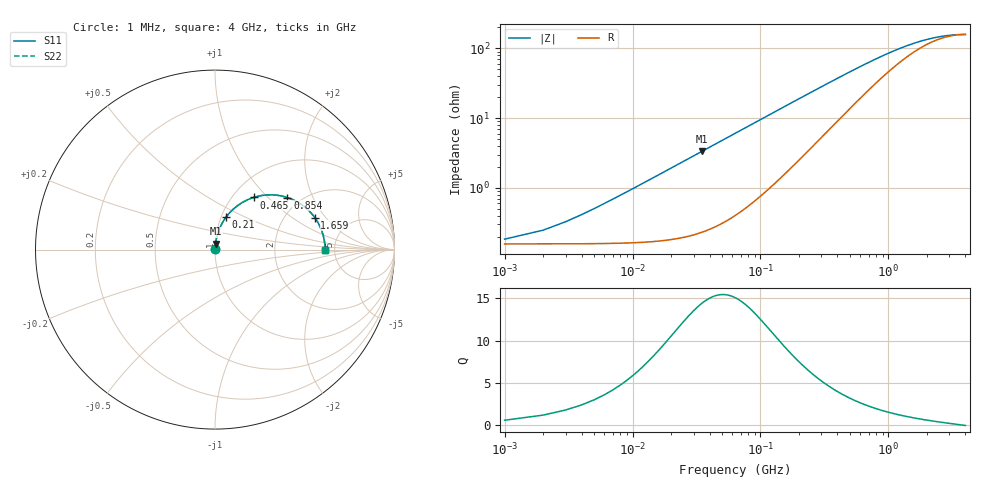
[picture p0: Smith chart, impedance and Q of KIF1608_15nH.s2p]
# MHz S RI R 50
!Freq ReS11 ImS11 ReS21 ImS21 ReS12 ImS12 ReS22 ImS22
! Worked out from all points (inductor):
!   4000 points, 1 MHz to 4 GHz, reference 50 ohm
!   read as one part in series: L = 15.2 nH near 21 MHz
!   highest Q = 14.4 at 35 MHz (marker M1), where L = 15.2 nH
!   self-resonance near 3.966 GHz
!   S11 on the Smith chart (normalised r, x): 1 MHz: 1.00, +0.00; 210 MHz: 1.05, +0.39; 465 MHz: 1.24, +0.83; 854 MHz: 1.71, +1.32; 1.659 GHz: 2.88, +1.56; 4 GHz: 4.17, -0.02
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1  0.00157 0.000954  0.9984 -0.000954  0.9984 -0.000954  0.00157 0.000954
11  0.00175 0.0105  0.9982 -0.0105  0.9982 -0.0105  0.00175 0.0105
24  0.00244 0.0229  0.9976 -0.0229  0.9976 -0.0229  0.00244 0.0229
29  0.00284 0.0276  0.9972 -0.0276  0.9972 -0.0276  0.00284 0.0276
35  0.00342 0.0333  0.9966 -0.0333  0.9966 -0.0333  0.00342 0.0333
46  0.00476 0.0436  0.9952 -0.0436  0.9952 -0.0436  0.00476 0.0436
60  0.00698 0.0567  0.993 -0.0567  0.993 -0.0567  0.00698 0.0567
77  0.0104 0.0723  0.9896 -0.0723  0.9896 -0.0723  0.0104 0.0723
96  0.0152 0.0894  0.9848 -0.0894  0.9848 -0.0894  0.0152 0.0894
146  0.0321 0.1321  0.9679 -0.1321  0.9679 -0.1321  0.0321 0.1321
210  0.0613 0.1804  0.9387 -0.1804  0.9387 -0.1804  0.0613 0.1804
321  0.1249 0.2443  0.8751 -0.2443  0.8751 -0.2443  0.1249 0.2443
465  0.2146 0.2905  0.7854 -0.2905  0.7854 -0.2905  0.2146 0.2905
668  0.3264 0.3046  0.6736 -0.3046  0.6736 -0.3046  0.3264 0.3046
854  0.4037 0.2898  0.5963 -0.2898  0.5963 -0.2898  0.4037 0.2898
1076  0.4685 0.2596  0.5315 -0.2596  0.5315 -0.2596  0.4685 0.2596
1334  0.5178 0.2218  0.4822 -0.2218  0.4822 -0.2218  0.5178 0.2218
1659  0.5559 0.1782  0.4441 -0.1782  0.4441 -0.1782  0.5559 0.1782
2001  0.5797 0.1392  0.4203 -0.1392  0.4203 -0.1392  0.5797 0.1392
2667  0.6028 0.0798  0.3972 -0.0798  0.3972 -0.0798  0.6028 0.0798
3334  0.6114 0.0347  0.3886 -0.0347  0.3886 -0.0347  0.6114 0.0347
4000  0.6134 -0.00169  0.3866 0.00169  0.3866 0.00169  0.6134 -0.00169
